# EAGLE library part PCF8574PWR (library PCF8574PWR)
Remote I/O Expander 20-Pin TSSOP Texas Instruments PCF8574PWR I/O Expander, 20-Pin TSSOP Source: Datasheet
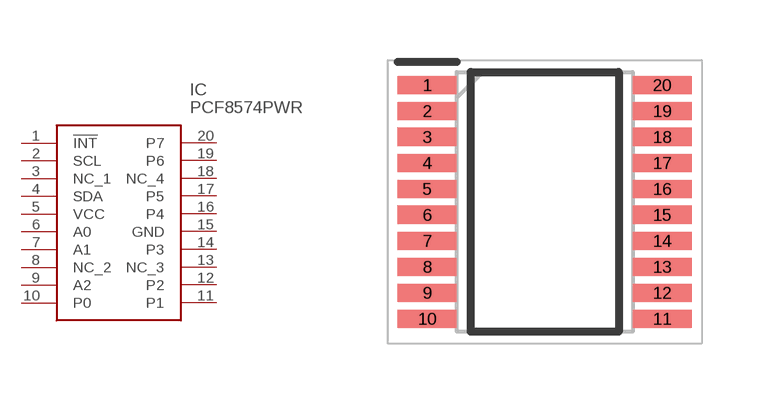
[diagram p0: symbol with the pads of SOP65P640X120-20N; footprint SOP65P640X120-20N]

Designator prefix IC

## PCF8574PWR (Description: Remote I/O Expander 20-Pin TSSOP Texas Instruments PCF8574PWR I/O Expander, 20-Pin TSSOP; Height: 1.2mm; Manufacturer_Name: Texas Instruments; Manufacturer_Part_Number: PCF8574PWR; Mouser_Part_Number: 595-PCF8574PWR; Mouser_Price-Stock: https://www.mouser.co.uk/ProductDetail/Texas-Instruments/PCF8574PWR?qs=X1HXWTtiZ0T3gnyuO%2Fq4CA%3D%3D)  [SOP65P640X120-20N]
1  !INT
2  SCL
3  NC_1
4  SDA
5  VCC
6  A0
7  A1
8  NC_2
9  A2
10  P0
11  P1
12  P2
13  NC_3
14  P3
15  GND
16  P4
17  P5
18  NC_4
19  P6
20  P7

## Footprint SOP65P640X120-20N (pad centres in mm)
PW (R-PDSO-G20)
smd 1.475 x 0.45: 1 -2.938,2.925; 2 -2.938,2.275; 3 -2.938,1.625; 4 -2.938,0.975; 5 -2.938,0.325; 6 -2.938,-0.325; 7 -2.938,-0.975; 8 -2.938,-1.625; 9 -2.938,-2.275; 10 -2.938,-2.925; 11 2.938,-2.925; 12 2.938,-2.275; 13 2.938,-1.625; 14 2.938,-0.975; 15 2.938,-0.325; 16 2.938,0.325; 17 2.938,0.975; 18 2.938,1.625; 19 2.938,2.275; 20 2.938,2.925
